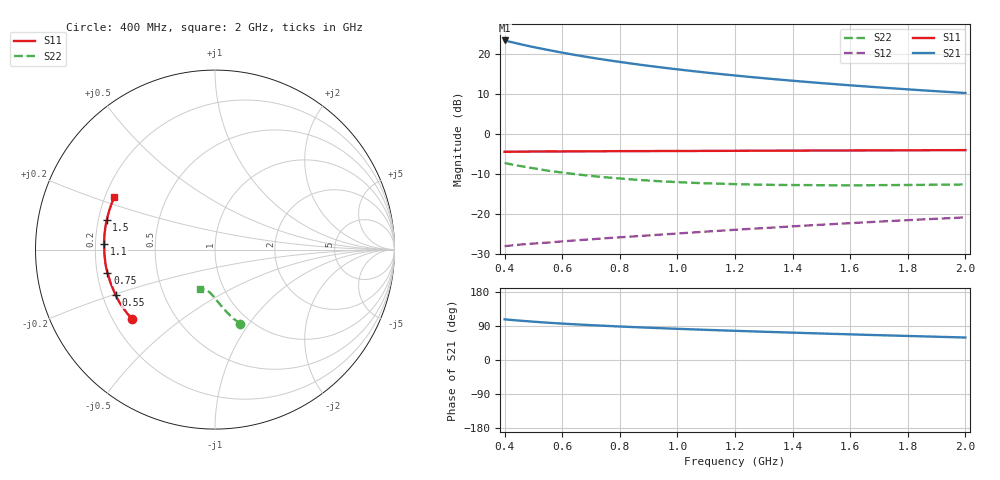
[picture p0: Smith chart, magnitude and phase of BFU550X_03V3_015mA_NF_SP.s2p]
! Filename:  P:\Prog\Test\Noise\ATS_data\Testdata_Net\bfu550X de embed 3currents\BFU550X_APG2013_44_C05_03p3V_015mA_NF_CM01_D.sf
! Date/Time: Mon 29/Jul/2013 14:56:12
! BFU550X_APG2013_44_C05_03p3V_1to35mA_NF_CM01_Bias6_R.sf
! Noise Parameter Data File
! BFU550X_APG2013_44_C05_03p3V_1to35mA_NF_CM01
! Date/time: Fri Jul 19 17:23:25 2013
! VAR V_out= 3.300000
! VAR I_out= 14.995000
! VAR V_in= 0.836000
! VAR I_in= 0.171300
! Device data file deembeded for feedlines and parallel
! Original file: \bfu550X de embed 3currents\BFU550X_APG2013_44_C05_03p3V_015mA_NF_CM01_R.sf
! Feed-files: PR005V01_100713_Feed1.s2p, PR005V01_100713_Feed2.s2p
! Parallel-file: PR005V01_100713_Par.s2p
# MHz S MA R 50
!  Freq-MHz  S11-mag  S11-arg  S21-mag  S21-arg  S12-mag  S12-arg  S22-mag  S22-arg
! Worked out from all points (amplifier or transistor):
!   37 points, 400 MHz to 2 GHz, reference 50 ohm
!   highest |S21| = 23.4 dB at 400 MHz (marker M1)
!   |S21| within 3 dB of that: start of sweep to 596.7 MHz
!   unconditionally stable (mu >= 1): 1.602 GHz to end of sweep
!   at 500 MHz: K = 0.55, MSG = 24.6 dB, |S12| = -27.3 dB
!   at 1.1 GHz: K = 0.89, MSG = 19.9 dB, |S12| = -24.3 dB
!   at 2 GHz: K = 1.04, MAG = 14.3 dB, |S12| = -20.8 dB
!   lowest NFmin = 0.88 dB at 480 MHz
!   S11 on the Smith chart (normalised r, x): 400 MHz: 0.28, -0.34; 550 MHz: 0.25, -0.21; 750 MHz: 0.24, -0.10; 1.1 GHz: 0.24, +0.02; 1.5 GHz: 0.23, +0.13; 2 GHz: 0.24, +0.23
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400  0.6036 -140.2  14.84 107.3  0.03991 43.8  0.4373 -71.3
420  0.6031 -142.5  14.24 106.0  0.04058 43.6  0.422 -72.8
440  0.6049 -144.8  13.71 104.7  0.0413 43.5  0.4083 -73.8
460  0.6058 -146.8  13.19 103.4  0.04195 43.3  0.3981 -75.2
500  0.6079 -150.7  12.28 101.1  0.04305 43.2  0.3754 -77.3
550  0.6093 -155.3  11.31 98.4  0.04422 43.4  0.35 -79.7
600  0.6089 -158.8  10.45 96.1  0.04579 43.7  0.3317 -81.8
650  0.6107 -162.2  9.708 93.9  0.04724 44.1  0.3152 -83.7
700  0.6111 -165.1  9.066 92.0  0.04862 44.5  0.3013 -85.4
750  0.6129 -167.9  8.498 90.2  0.05014 45.0  0.2897 -87.1
800  0.6147 -170.5  8.002 88.4  0.0515 45.4  0.2797 -88.7
850  0.6154 -172.9  7.554 86.8  0.05289 46.0  0.2709 -90.1
900  0.6153 -175.2  7.15 85.2  0.05439 46.6  0.2635 -91.4
950  0.6164 -177.2  6.792 83.7  0.05593 47.0  0.2573 -92.6
1000  0.6168 -179.2  6.465 82.3  0.05747 47.5  0.252 -93.8
1100  0.6188 177.1  5.893 79.6  0.0607 48.4  0.2437 -96.0
1200  0.6204 173.8  5.416 77.0  0.06391 49.2  0.2379 -98.0
1350  0.623 169.0  4.825 73.4  0.06887 50.2  0.2323 -100.8
1500  0.6253 164.8  4.352 69.9  0.07397 50.9  0.2306 -103.2
1600  0.6267 162.1  4.084 67.7  0.07738 51.3  0.2299 -104.8
1750  0.6287 158.2  3.737 64.5  0.08262 51.7  0.2315 -107.2
2000  0.6331 152.3  3.272 59.3  0.09139 52.0  0.2358 -110.7
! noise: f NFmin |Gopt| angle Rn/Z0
400  0.9598  0.1916  -176.6  0.0803
460  0.9439  0.2341  -176.1  0.0668
600  0.8971  0.2496  -176.9  0.0695
800  0.9498  0.2858  -175.6  0.0598
1000  0.9579  0.315  -175.9  0.0553
1200  0.9934  0.3393  -173.2  0.0535
1400  1.018  0.37  -168.6  0.0526
1600  1.138  0.339  -162.8  0.0649
1800  1.073  0.3898  -167.4  0.0515
2000  1.106  0.3922  -161.2  0.0638
